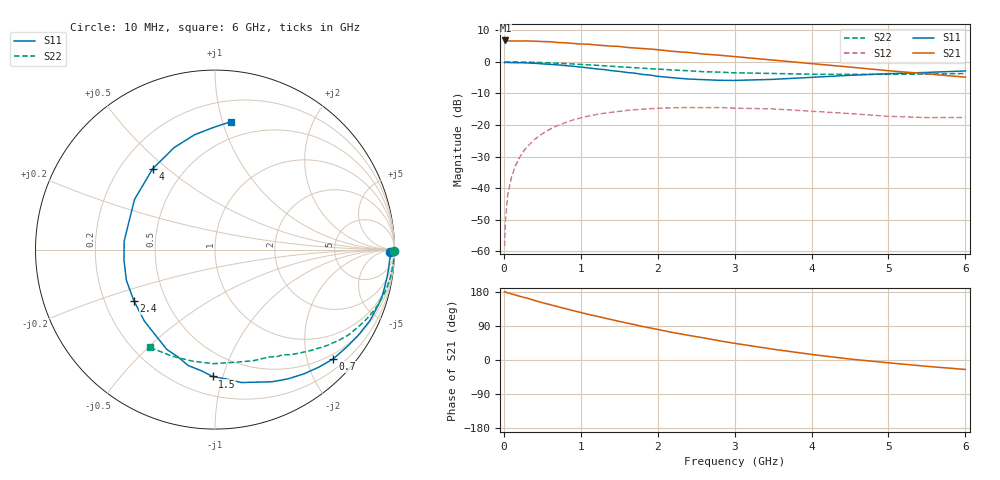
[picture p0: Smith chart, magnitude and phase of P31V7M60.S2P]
! SIEMENS Small Signal Semiconductors
! BFP181
! Si NPN RF Bipolar Junction Transistor in SOT143
! VCE = 1.75 V  IC = 0.6 mA
! Common Emitter S-Parameters:  March  1996
# GHz  S  MA  R  50
!  f  S11  S21  S12  S22
! GHz  MAG  ANG  MAG  ANG  MAG  ANG  MAG  ANG
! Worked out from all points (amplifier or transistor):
!   36 points, 10 MHz to 6 GHz, reference 50 ohm
!   highest |S21| = 6.8 dB at 20 MHz (marker M1)
!   |S21| within 3 dB of that: start of sweep to 2.025 GHz
!   unconditionally stable (mu >= 1): 3.575 GHz to end of sweep
!   at 250 MHz: K = 0.08, MSG = 17.6 dB, |S12| = -28.5 dB
!   at 1.4 GHz: K = 0.45, MSG = 10.5 dB, |S12| = -16.0 dB
!   at 6 GHz: K = 1.41, MAG = 2.6 dB, |S12| = -17.6 dB
!   S11 on the Smith chart (normalised r, x): 10 MHz: 58, -37; 700 MHz: 0.40, -2.50; 1.5 GHz: 0.33, -0.93; 2.4 GHz: 0.33, -0.26; 4 GHz: 0.34, +0.45; 6 GHz: 0.36, +1.07
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0.01  0.9756 -0.9  2.172 179.8  0.0012 91.0  0.9991 -0.3
0.02  0.9842 -1.4  2.185 179.5  0.0029 90.4  0.9976 -0.6
0.05  0.9754 -2.9  2.16 177.3  0.0078 89.8  0.9975 -1.5
0.1  0.9734 -6.2  2.145 174.4  0.015 84.3  0.9984 -2.9
0.2  0.968 -12.3  2.149 168.6  0.03 81.6  0.994 -5.9
0.3  0.9613 -18.6  2.151 163.4  0.0448 77.0  0.9899 -8.9
0.4  0.9496 -24.6  2.127 157.1  0.0592 73.2  0.9831 -11.8
0.6  0.9123 -36.6  2.087 146.1  0.0858 64.3  0.9639 -17.4
0.7  0.8969 -42.8  2.026 140.7  0.0979 60.4  0.9523 -20.2
0.9  0.8514 -54.4  1.962 130.3  0.1199 52.7  0.9255 -25.2
1.1  0.8024 -66.6  1.906 120.3  0.1385 45.4  0.8965 -30.0
1.5  0.7069 -91.1  1.758 101.9  0.1647 32.3  0.8353 -38.6
1.8  0.632 -109.2  1.629 88.5  0.1782 24.4  0.7939 -43.9
2.2  0.5602 -134.6  1.466 72.4  0.1871 14.3  0.7439 -50.8
2.4  0.5344 -147.7  1.409 65.1  0.1889 9.7  0.7228 -54.1
2.8  0.5104 -173.6  1.275 50.8  0.1887 2.2  0.6885 -60.0
3  0.5082 174.6  1.213 44.0  0.1852 -1.5  0.67 -63.2
3.5  0.5283 148.0  1.067 28.5  0.1796 -8.3  0.6548 -71.1
4  0.5685 127.7  0.938 14.7  0.1649 -13.5  0.6368 -80.5
4.5  0.6123 111.8  0.827 2.5  0.1514 -17.1  0.6357 -90.9
5.5  0.6808 90.7  0.646 -16.7  0.1312 -13.0  0.6408 -112.5
6  0.7182 82.9  0.573 -25.0  0.1313 -9.7  0.6544 -123.7
